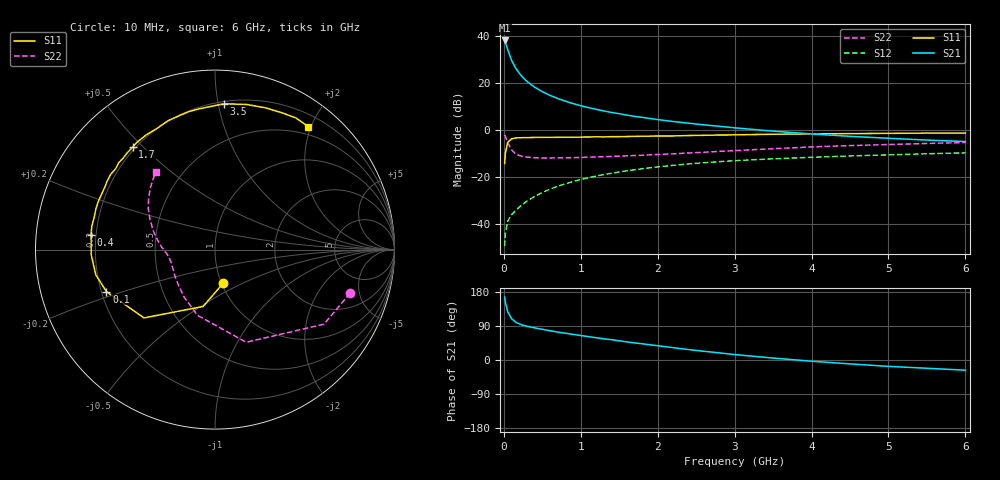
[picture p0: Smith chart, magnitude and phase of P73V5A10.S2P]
! SIEMENS Small Signal Semiconductors
! BFP196
! Si NPN RF Bipolar Junction Transistor in SOT143
! VCE = 3.5 V  IC = 100 mA
! Common Emitter S-Parameters:  May  1996
# GHz  S  MA  R  50
!  f  S11  S21  S12  S22
! GHz  MAG  ANG  MAG  ANG  MAG  ANG  MAG  ANG
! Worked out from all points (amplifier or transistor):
!   36 points, 10 MHz to 6 GHz, reference 50 ohm
!   highest |S21| = 38.1 dB at 10 MHz (marker M1)
!   |S21| within 3 dB of that: start of sweep to 41.84 MHz
!   unconditionally stable (mu >= 1): 315.8 MHz to 4.929 GHz
!   at 250 MHz: K = 0.95, MSG = 26.9 dB, |S12| = -31.5 dB
!   at 1.4 GHz: K = 1.09, MAG = 11.1 dB, |S12| = -18.4 dB
!   at 6 GHz: K = 0.99, MSG = 2.4 dB, |S12| = -9.7 dB
!   S11 on the Smith chart (normalised r, x): 10 MHz: 1.02, -0.40; 100 MHz: 0.22, -0.18; 400 MHz: 0.18, +0.06; 1.7 GHz: 0.19, +0.47; 3.5 GHz: 0.22, +1.04; 6 GHz: 0.37, +1.95
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0.01  0.1935 -76.6  80.09 165.9  0.0034 74.3  0.7909 -17.9
0.02  0.3236 -101.8  73.26 152.5  0.0063 68.7  0.7357 -34.4
0.05  0.5489 -136.1  51.52 127.4  0.0115 54.7  0.5446 -71.4
0.1  0.6484 -158.8  30.51 109.0  0.0158 53.1  0.3792 -104.8
0.15  0.6786 -168.0  21.16 100.4  0.0192 55.0  0.3154 -123.0
0.2  0.6837 -173.9  16.12 95.4  0.023 58.4  0.2874 -134.3
0.25  0.6907 -177.9  12.9 91.8  0.0266 60.8  0.2726 -142.5
0.3  0.69 179.0  10.79 89.1  0.0309 63.2  0.2656 -147.9
0.4  0.6954 173.1  8.157 84.8  0.0389 65.4  0.2575 -155.6
0.5  0.6986 169.4  6.532 81.0  0.0468 66.4  0.2549 -160.5
0.6  0.6968 165.1  5.454 77.2  0.0556 66.7  0.2551 -163.8
0.7  0.7011 161.2  4.682 73.6  0.0636 66.3  0.2559 -166.3
0.9  0.7031 154.3  3.646 67.6  0.0806 64.5  0.2585 -170.2
1.1  0.7118 147.6  2.999 61.6  0.0966 62.3  0.2648 -173.0
1.3  0.7138 140.8  2.544 55.9  0.1131 59.7  0.2707 -175.5
1.7  0.7324 128.8  1.948 45.0  0.1431 53.8  0.2867 179.6
2.2  0.7488 115.5  1.517 32.6  0.1776 45.8  0.3117 173.6
2.8  0.7826 100.6  1.201 18.8  0.2127 36.6  0.3518 164.7
3.5  0.8143 86.4  0.946 5.1  0.2446 26.4  0.4007 154.8
4.5  0.8385 70.4  0.734 -10.3  0.2813 14.3  0.4662 142.5
5.5  0.861 58.4  0.611 -21.8  0.3126 3.4  0.5184 132.3
6  0.8597 52.9  0.57 -26.9  0.3273 -2.3  0.5428 127.3
